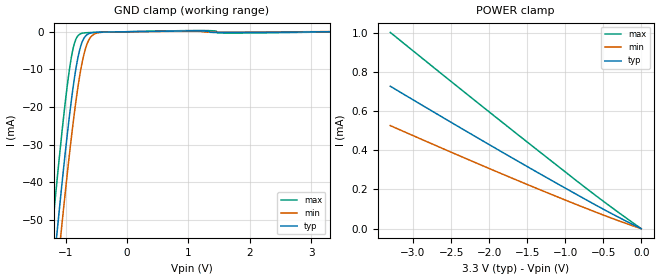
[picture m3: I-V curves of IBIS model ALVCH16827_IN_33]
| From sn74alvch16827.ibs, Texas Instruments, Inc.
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[Model]   ALVCH16827_IN_33
Model_type  Input
Vinl=0.8
Vinh=2.0
| variable   typ   min   max
C_comp   1.96pF   1.60pF   2.29pF
[Temperature Range]   40   100   -40
| Ambient temperature   25   85   -40
[Voltage range]   3.3   3   3.6
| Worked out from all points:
|   GND clamp passes 1 mA (typ) near -0.67 V on its own axis
[GND Clamp]
| ALVCH16827_IN_33
|   Voltage   I(typ)   I(min)   I(max)
-3.3V     -452.3mA   -460.9mA   -441.9mA
-1.225V   -67.1mA    -77.86mA   -53.3mA
-1.14V    -52.86mA   -63.63mA   -39mA
-1.07V    -41.56mA   -52.27mA   -27.81mA
-985mV    -28.62mA   -39.07mA   -15.5mA
-905mV    -17.69mA   -27.53mA   -6.417mA
-845mV    -10.81mA   -19.7mA    -2.393mA
-765mV    -4.304mA   -10.92mA   -590.3uA
-705mV    -1.763mA   -6.058mA   -327.5uA
-635mV    -595.1uA   -2.555mA   -248.5uA
-470mV    -136.5uA   -260.9uA   -175uA
3.3V      1.116nA    40.72uA    -79.23uA
[POWER Clamp]
| ALVCH16827_IN_33
|   Voltage   I(typ)   I(min)   I(max)
-3.3V     726.6uA    525.8uA    1.001mA
-1.955V   418.9uA    299.7uA    582uA
-845mV    173.4uA    122.2uA    242.6uA
-430mV    85.18uA    59.42uA    120.2uA
-48.03fV  1.116nA    59.61nA    9.389pA
